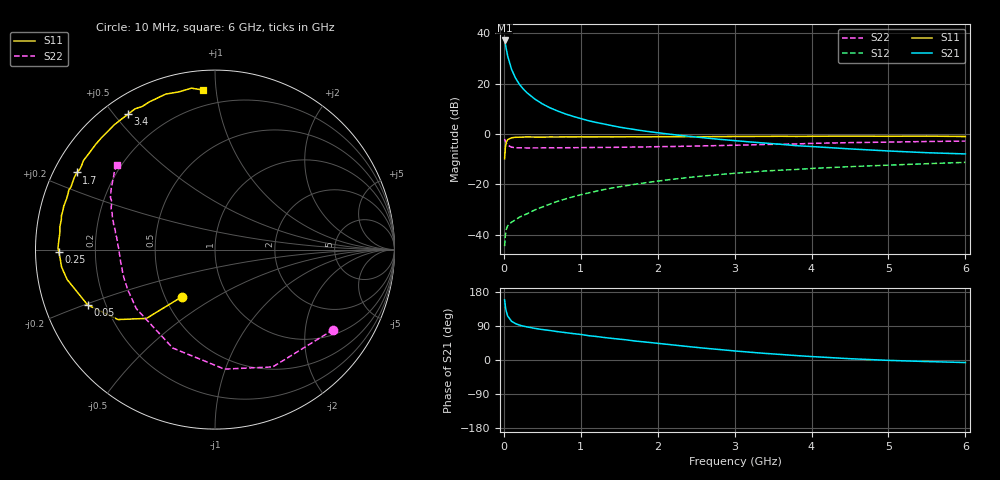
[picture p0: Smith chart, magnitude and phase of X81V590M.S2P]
! SIEMENS Small Signal Semiconductors
! BFP136W
! Si NPN RF Bipolar Junction Transistor in SOT343
! VCE = 1.5 V  IC = 90 mA
! Common Emitter S-Parameters:  September  1994
# GHz  S  MA  R  50
!  f  S11  S21  S12  S22
! GHz  MAG  ANG  MAG  ANG  MAG  ANG  MAG  ANG
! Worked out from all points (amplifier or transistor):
!   40 points, 10 MHz to 6 GHz, reference 50 ohm
!   highest |S21| = 37.2 dB at 10 MHz (marker M1)
!   |S21| within 3 dB of that: start of sweep to 29.3 MHz
!   unconditionally stable (mu >= 1): 464.8 MHz to 2.976 GHz; 3.797216 GHz to 3.803546 GHz
!   at 200 MHz: K = 0.69, MSG = 26.5 dB, |S12| = -33.1 dB
!   at 1.5 GHz: K = 1.11, MAG = 9.8 dB, |S12| = -21.0 dB
!   at 6 GHz: K = 1.00, MSG = 1.7 dB, |S12| = -11.3 dB
!   S11 on the Smith chart (normalised r, x): 10 MHz: 0.61, -0.36; 50 MHz: 0.13, -0.20; 250 MHz: 0.07, -0.01; 1.7 GHz: 0.07, +0.26; 3.4 GHz: 0.07, +0.54; 6 GHz: 0.11, +0.92
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0.01  0.3229 -125.2  72.35 158.7  0.0059 68.1  0.7959 -34.1
0.02  0.5412 -134.9  61.18 141.6  0.0098 53.7  0.7285 -63.8
0.03  0.6664 -144.2  50.54 129.8  0.0125 46.6  0.6679 -85.5
0.05  0.7737 -156.5  35.43 116.0  0.015 37.0  0.5968 -113.2
0.1  0.8407 -168.6  19.34 102.2  0.0177 34.9  0.5481 -143.1
0.15  0.8605 -173.6  13.11 96.1  0.0197 38.4  0.5349 -155.0
0.2  0.8639 -176.6  9.834 92.3  0.0221 40.9  0.5317 -161.4
0.25  0.8703 -179.2  7.931 89.5  0.024 44.3  0.5307 -165.5
0.3  0.875 179.4  6.627 87.5  0.0259 47.7  0.5288 -168.2
0.4  0.8711 176.1  4.991 83.6  0.0309 52.1  0.53 -171.9
0.5  0.8693 173.5  3.977 80.4  0.0354 55.3  0.5305 -174.4
0.6  0.8735 171.5  3.318 77.8  0.0405 57.5  0.5312 -176.1
0.7  0.8721 169.0  2.862 74.8  0.046 59.4  0.5332 -177.4
0.9  0.875 165.7  2.243 69.7  0.0566 60.7  0.5349 -179.8
1.1  0.8741 161.4  1.839 64.2  0.0673 61.4  0.5386 178.5
1.7  0.8815 150.8  1.227 50.2  0.1001 59.0  0.5505 173.5
2.2  0.8833 142.6  0.974 39.7  0.1263 55.2  0.5645 169.6
3.2  0.8944 125.6  0.696 20.6  0.1746 45.4  0.6075 160.6
3.4  0.8965 122.7  0.66 17.4  0.1844 43.2  0.6206 158.8
4.5  0.9089 107.6  0.506 3.4  0.2246 32.8  0.6742 148.9
5.5  0.9091 98.3  0.425 -4.1  0.2571 24.7  0.7101 142.1
6  0.891 94.2  0.402 -6.7  0.2731 20.4  0.7231 139.1
